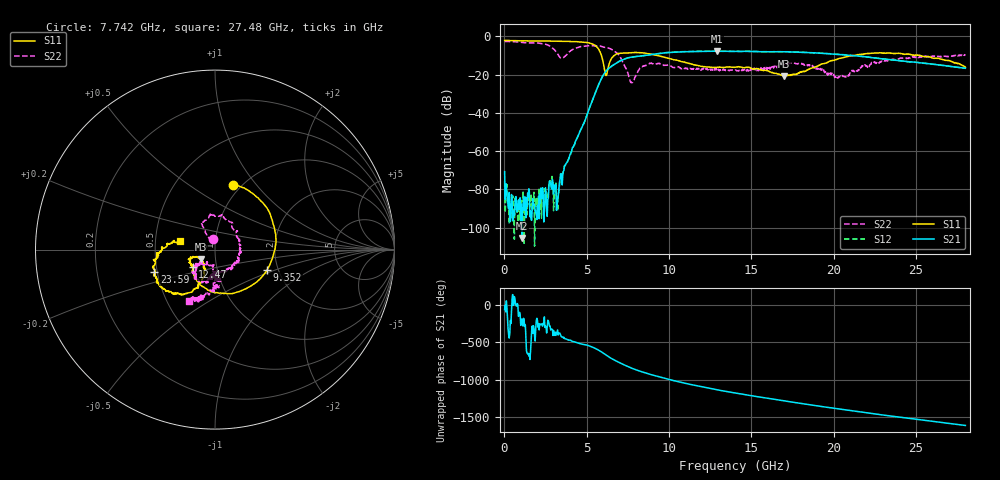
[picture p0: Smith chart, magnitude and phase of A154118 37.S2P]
!  2-Port S-parameters saved by WinCal
! VAR MeasName=S-Parameters (CALIBRATED_DATA) read from VNA (N5230A)
! VAR MeasDate=2015-9-10 14:37:17
! VAR NAME=A154118 37
! VAR FILENAME=A154118 37.S2P
! VAR DATE=2015-9-10 14:37:17
! VAR PHYS_PORTS=1,2
# Hz S DB R 50
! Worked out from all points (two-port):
!   801 points, 10 MHz to 28 GHz, reference 50 ohm
!   highest |S21| = -7.75 dB at 12.89 GHz (marker M1); lowest = -105.3 dB at 1.06 GHz (marker M2)
!   |S21| within 3 dB of the highest: 7.828 GHz to 22.02 GHz (14.19 GHz wide, 95.1 % of centre)
!   lowest |S11| = -20.6 dB at 16.98 GHz (marker M3), VSWR 1.20, Z = 42.7 - j4.59 ohm
!   |S11| at or under -10 dB: 5.891 GHz to 6.667 GHz (776.5 MHz wide, 12.4 % of centre); 9.275 GHz to 21.23 GHz (11.95 GHz wide, 78.4 % of centre); 25.26 GHz to end of sweep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
!   |S22| runs from -24.2 to -2.7 dB; largest |S21 - S12| = 0.0089
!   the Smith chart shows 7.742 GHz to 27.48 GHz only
!   S11 on the Smith chart (normalised r, x): 7.742 GHz: 0.91, +0.77; 9.352 GHz: 1.75, -0.44; 12.47 GHz: 0.76, -0.15; 23.59 GHz: 0.48, -0.14; 27.48 GHz: 0.67, +0.07
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1e7  -2.15 179.7  -70.66 -58.8  -75.77 -41.7  -2.67 179.8
1.059625e9  -2.34 165.7  -105.32 176.2  -85.66 -144.2  -3.16 153.9
2.5291e9  -2.46 145.9  -83.40 66.9  -81.11 55.6  -4.18 100.5
3.193862e9  -2.51 134.9  -89.25 -0.5  -83.00 -36.2  -8.71 25.7
3.753662e9  -2.59 123.8  -66.35 -95.1  -66.57 -85.2  -9.81 -108.7
4.698325e9  -3.01 98.2  -47.67 -161.3  -47.51 -161.5  -5.29 166.3
5.642988e9  -5.81 38.4  -26.89 126.0  -26.84 126.3  -5.00 123.4
6.097825e9  -18.38 -59.0  -18.96 61.5  -18.89 61.4  -5.77 103.5
6.552662e9  -10.97 141.3  -15.35 -1.3  -15.28 -1.5  -7.04 81.9
7.742238e9  -8.52 74.5  -10.84 -125.7  -10.83 -125.9  -24.23 100.6
9.351662e9  -10.12 -21.4  -9.09 121.8  -9.01 121.8  -14.14 79.4
1.110104e10  -13.92 -120.1  -8.00 26.5  -7.92 25.9  -16.69 20.2
1.246555e10  -15.97 -141.9  -7.81 -35.5  -7.76 -36.2  -17.64 -40.0
1.28854e10  -16.18 -144.8  -7.75 -53.0  -7.72 -53.7  -16.95 -53.0
1.4005e10  -16.09 -151.9  -7.88 -96.9  -7.86 -97.5  -17.80 -82.6
1.697894e10  -20.63 -145.1  -8.01 157.9  -8.03 157.5  -14.65 -106.5
1.869332e10  -16.44 -113.0  -8.56 100.6  -8.56 100.0  -15.26 -131.0
2.019779e10  -11.99 -118.7  -9.46 52.1  -9.35 51.1  -21.44 -123.4
2.334666e10  -8.73 -156.9  -12.08 -42.8  -12.04 -44.0  -12.79 -94.2
2.359158e10  -8.88 -159.9  -12.34 -49.5  -12.36 -50.4  -11.95 -98.3
2.747519e10  -13.87 166.7  -16.14 -157.5  -16.12 -158.5  -9.87 -116.6
2.8e10  -16.13 167.6  -16.68 -172.4  -16.69 -173.4  -9.38 -117.3
